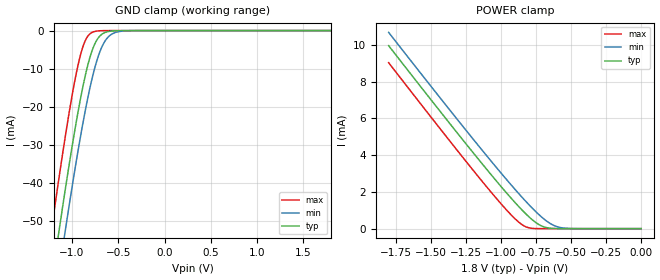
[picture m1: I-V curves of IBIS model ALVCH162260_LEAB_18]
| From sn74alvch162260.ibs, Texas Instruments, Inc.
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[Model]   ALVCH162260_LEAB_18
Model_type  Input
Vinl=0.5775
Vinh=1.2675
| variable   typ   min   max
C_comp   1.72pF   1.57pF   2.08pF
[Temperature Range]   40   100   -40
| Ambient temperature   25   85   -40
[Voltage range]   1.8   1.65   1.95
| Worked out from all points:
|   GND clamp passes 1 mA (typ) near -0.68 V on its own axis
|   POWER clamp passes 1 mA (typ) near -0.85 V on its own axis
[GND Clamp]
| ALVCH162260_LEAB_18
|   Voltage   I(typ)   I(min)   I(max)
-1.8V     -169.5mA   -179.7mA   -156.7mA
-1.245V   -70.18mA   -81.02mA   -56.25mA
-1.22V    -65.92mA   -76.78mA   -51.96mA
-1.14V    -52.55mA   -63.42mA   -38.55mA
-1.075V   -42.06mA   -52.87mA   -28.16mA
-920mV    -19.37mA   -29.44mA   -7.486mA
-860mV    -12.16mA   -21.41mA   -2.808mA
-795mV    -6.112mA   -13.8mA    -645.2uA
-730mV    -2.404mA   -7.745mA   -117.8uA
-660mV    -692.8uA   -3.429mA   -17.66uA
-495mV    -25.94uA   -271uA     -195.5nA
1.8V      1.111nA    770.5nA    2.881pA
[POWER Clamp]
| ALVCH162260_LEAB_18
|   Voltage   I(typ)   I(min)   I(max)
-1.8V     9.965mA    10.69mA    9.037mA
-1.38V    5.878mA    6.614mA    4.929mA
-1.105V   3.269mA    4.008mA    2.314mA
-940mV    1.776mA    2.501mA    856.4uA
-885mV    1.307mA    2.018mA    440uA
-845mV    982.9uA    1.676mA    200.1uA
-795mV    611.2uA    1.266mA    38.41uA
-715mV    166.7uA    670.1uA    941.7nA
-645mV    22.22uA    268.3uA    31.48nA
-585mV    2.717uA    77.14uA    1.709nA
-485mV    73.51nA    4.604uA    18.27pA
-16.28fV  3.324pA    5.122pA    3.398pA
